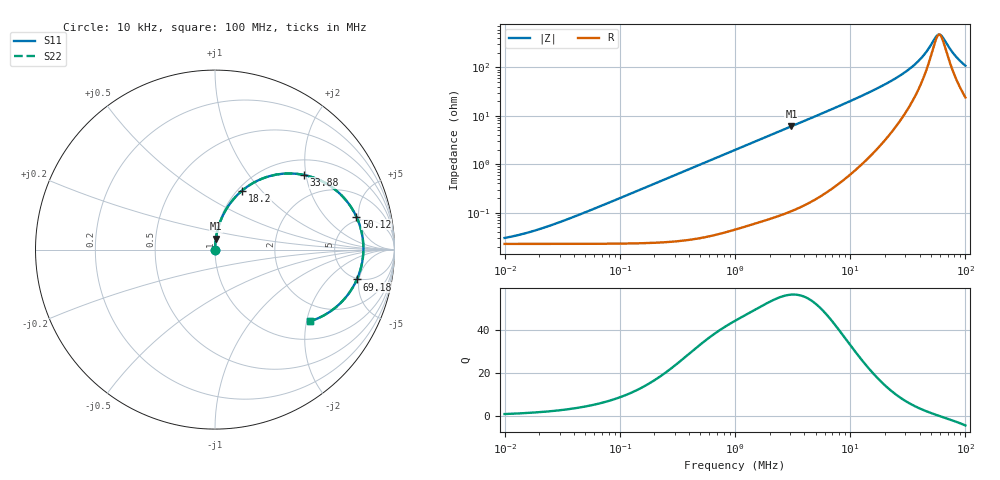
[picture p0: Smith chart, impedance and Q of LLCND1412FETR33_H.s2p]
! LLCND1412FETR33_H  S-PARAMETER MODEL  ( Standard Model )
! Model Generated by TAIYO YUDEN Corporation (http://www.ty-top.com)
! Version 1.0
! TAIYO YUDEN Control No. 241002
! Copyright(c) 2024 TAIYO YUDEN CO.,LTD. All Rights Reserved.
! Product Description (link to TY-COMPAS)
! https://ds.yuden.co.jp/TYCOMPAS/or/detail?pn=LLCND1412FETR33MH&u=M
! Products Name : Inductors
! Characteristics :
!  Inductance : 0.33 [uH] , SRF(min) : - [Hz] , DC Resistance(max) : 25 [mOhm]
!  Rated Current : Saturation  3.6 [A] (dL = 30 [%]), Temp Rise  4.2 [A] (dT = 40 [degC])
!  Case Size : 1.4 x 1.2 / 0.055 x 0.047 [mm/inch] , Thickness : 0.65 / 0.026 [mm/inch]
!  (Conditions: Temperature = 25 [degC] , DC Bias Current = 0 [A])
! External Node Assignments :
!  1  o---GGG---o  2
! GND o---------o GND
! Frequency Range : 10kHz  -  100MHz  [ 402 STEP ]
# MHz S RI R 50
! Freq[MHz].  S11 Real  S11 Imag  S21 Real  S21 Imag  S12 Real  S12 Imag  S22 Real  S22 Imag
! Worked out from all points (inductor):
!   401 points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, 10 kHz to 100 MHz, reference 50 ohm
!   read as one part in series: L = 315 nH near 34.67 kHz
!   highest Q = 56.2 at 3.09 MHz (marker M1), where L = 311 nH
!   self-resonance near 59.33 MHz
!   S11 on the Smith chart (normalised r, x): 10 kHz: 1.00, +0.00; 18.2 MHz: 1.05, +0.79; 33.88 MHz: 1.36, +1.95; 50.12 MHz: 4.39, +4.66; 69.18 MHz: 4.86, -4.65; 100 MHz: 1.48, -2.11
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0.01  0.000226 0.000198  0.9998 -0.000198  0.9998 -0.000198  0.000226 0.000198
0.019498  0.000226 0.000385  0.9998 -0.000385  0.9998 -0.000385  0.000226 0.000385
0.046774  0.000227 0.000924  0.9998 -0.000924  0.9998 -0.000924  0.000227 0.000924
0.218776  0.00026 0.00432  0.9997 -0.00432  0.9997 -0.00432  0.00026 0.00432
1  0.00083 0.0196  0.9992 -0.0196  0.9992 -0.0196  0.00083 0.0196
3.090295  0.00469 0.06  0.9953 -0.06  0.9953 -0.06  0.00469 0.06
4.677351  0.00999 0.0905  0.99 -0.0905  0.99 -0.0905  0.00999 0.0905
10.71519  0.0507 0.2037  0.9493 -0.2037  0.9493 -0.2037  0.0507 0.2037
18.19701  0.1494 0.3272  0.8506 -0.3272  0.8506 -0.3272  0.1494 0.3272
21.87762  0.2176 0.3742  0.7824 -0.3742  0.7824 -0.3742  0.2176 0.3742
28.18383  0.3581 0.4205  0.6419 -0.4205  0.6419 -0.4205  0.3581 0.4205
33.88442  0.4966 0.4157  0.5034 -0.4157  0.5034 -0.4157  0.4966 0.4157
41.68694  0.6677 0.3356  0.3323 -0.3356  0.3323 -0.3356  0.6677 0.3356
45.70882  0.7351 0.2686  0.2649 -0.2686  0.2649 -0.2686  0.7351 0.2686
50.11872  0.7876 0.1837  0.2124 -0.1837  0.2124 -0.1837  0.7876 0.1837
54.95409  0.8192 0.0859  0.1808 -0.0859  0.1808 -0.0859  0.8192 0.0859
58.88437  0.8269 0.00827  0.1731 -0.00827  0.1731 -0.00827  0.8269 0.00827
63.09573  0.8202 -0.0692  0.1798 0.0692  0.1798 0.0692  0.8202 -0.0692
69.1831  0.7905 -0.1663  0.2095 0.1663  0.2095 0.1663  0.7905 -0.1663
75.85776  0.7408 -0.2506  0.2592 0.2506  0.2592 0.2506  0.7408 -0.2506
83.17638  0.6771 -0.318  0.3229 0.318  0.3229 0.318  0.6771 -0.318
100  0.5317 -0.3984  0.4683 0.3984  0.4683 0.3984  0.5317 -0.3984
